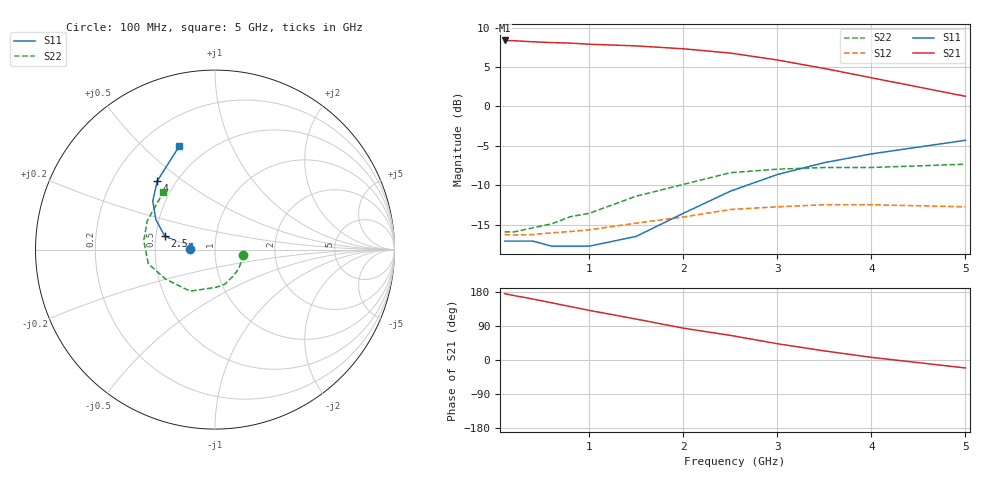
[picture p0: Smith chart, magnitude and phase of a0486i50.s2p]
!  MSA-0486 S AND NOISE PARAMETERS
!  Id=50mA  LAST UPDATED 07-22-92
# ghz s ma r 50
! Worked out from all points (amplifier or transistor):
!   13 points, 100 MHz to 5 GHz, reference 50 ohm
!   highest |S21| = 8.4 dB at 100 MHz (marker M1)
!   |S21| within 3 dB of that: start of sweep to 3.243 GHz
!   unconditionally stable (mu >= 1): start of sweep to 2.809 GHz; 3.755 GHz to end of sweep
!   at 400 MHz: K = 1.38, MAG = 8.5 dB, |S12| = -16.2 dB
!   at 1.5 GHz: K = 1.23, MAG = 8.3 dB, |S12| = -14.8 dB
!   at 5 GHz: K = 1.05, MAG = 5.7 dB, |S12| = -12.7 dB
!   lowest NFmin = 6.70 dB at 100 MHz
!   S11 on the Smith chart (normalised r, x): 100 MHz: 0.75, +0.01; 2.5 GHz: 0.56, +0.09; 4 GHz: 0.40, +0.40; 5 GHz: 0.35, +0.65
0.1  0.14 178.0  2.62 175.0  0.154 1.0  0.16 -10.0
0.2  0.14 175.0  2.61 170.0  0.153 2.0  0.16 -20.0
0.4  0.14 171.0  2.57 161.0  0.154 3.0  0.17 -39.0
0.6  0.13 168.0  2.54 151.0  0.158 4.0  0.18 -57.0
0.8  0.13 166.0  2.52 141.0  0.161 5.0  0.2 -74.0
1  0.13 165.0  2.48 131.0  0.165 6.0  0.21 -88.0
1.5  0.15 168.0  2.42 108.0  0.182 8.0  0.27 -121.0
2  0.21 168.0  2.32 84.0  0.199 7.0  0.32 -149.0
2.5  0.29 165.0  2.18 65.0  0.222 4.0  0.38 -168.0
3  0.37 153.0  1.97 43.0  0.231 -1.0  0.4 173.0
3.5  0.44 142.0  1.74 24.0  0.238 -5.0  0.41 157.0
4  0.5 130.0  1.52 7.0  0.238 -10.0  0.41 145.0
5  0.61 109.0  1.16 -21.0  0.231 -17.0  0.43 132.0
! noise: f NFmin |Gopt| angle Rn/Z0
0.1  6.7  0.12  -179  0.65
0.5  6.7  0.13  -176  0.65
1  7  0.14  -170  0.65
2  7.7  0.2  -154  0.65
